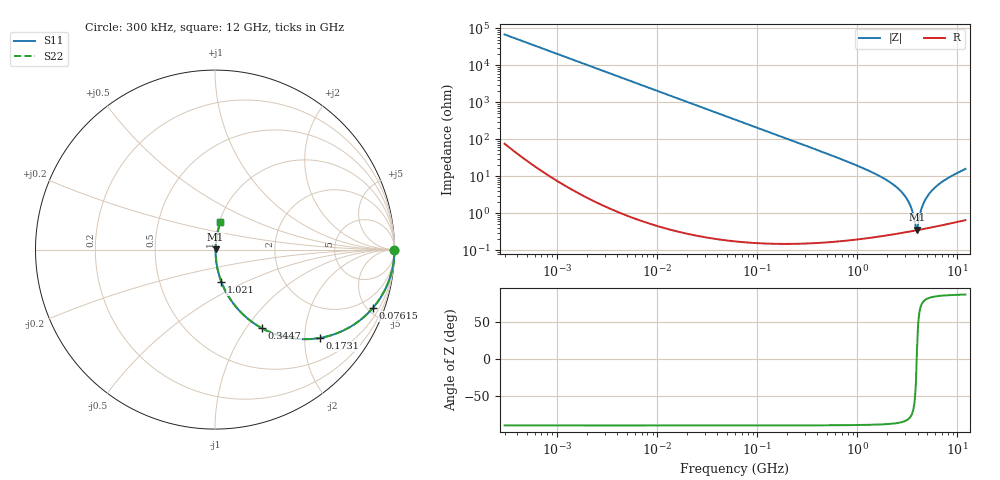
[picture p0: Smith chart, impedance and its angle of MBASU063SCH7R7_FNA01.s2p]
! MBASU063SCH7R7_FNA01  S-PARAMETER MODEL  ( General Type )
! Model Generated by TAIYO YUDEN Corporation (http://www.ty-top.com)
! Version 1.0
! TAIYO YUDEN Control No. 130801
! Copyright(c) 2013 TAIYO YUDEN CO.,LTD. All Rights Reserved.
! Product Description (link to TY-COMPAS)
! https://ds.yuden.co.jp/TYCOMPAS/or/detail?pn=MBASU063SCH7R7DFNA01&u=M
! Products Name : Multilayer Ceramic Capacitors
! Characteristics :
!  Capacitance : 7.7 pF , Rated Voltage : 50V , TCC : CH / C0H
!  Case Size : 0.6 x 0.3 / 0.024 x 0.012 [mm/inch] , Thickness : 0.3 / 0.012 [mm/inch]
!  (Conditions: Temperature = 25 degC , DC Bias Current/Voltage = 0A / 0V)
! External Node Assignments :
!  1  o---| |---o  2
! GND o---------o GND
! Frequency Range : 0.3MHz  -  12000MHz  [ 401 STEP ]
# MHz S RI R 50
! Freq[MHz].  S11 Real  S11 Imag  S21 Real  S21 Imag  S12 Real  S12 Imag  S22 Real  S22 Imag
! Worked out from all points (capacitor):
!   401 points, 300 kHz to 12 GHz, reference 50 ohm
!   read as one part in series: C = 7.73 pF near 316.3 kHz
!   lowest |Z| = 356 mohm at 3.944 GHz (marker M1)
!   series resonance near 3.917 GHz, so ESL is about 210 pH
!   S11 on the Smith chart (normalised r, x): 300 kHz: open; 76.15 MHz: 1.00, -5.41; 173.1 MHz: 1.00, -2.38; 344.7 MHz: 1.00, -1.19; 1.021 GHz: 1.00, -0.38; 12 GHz: 1.01, +0.32
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0.3  1 -0.00146  3.72e-06 0.00146  3.72e-06 0.00146  1 -0.00146
1.769972  0.9999 -0.00859  7.61e-05 0.00859  7.61e-05 0.00859  0.9999 -0.00859
10.44266  0.9974 -0.0506  0.00257 0.0506  0.00257 0.0506  0.9974 -0.0506
27.10171  0.9829 -0.1293  0.0171 0.1293  0.0171 0.1293  0.9829 -0.1293
60  0.9217 -0.2685  0.0783 0.2685  0.0783 0.2685  0.9217 -0.2685
76.15486  0.8796 -0.3252  0.1204 0.3252  0.1204 0.3252  0.8796 -0.3252
173.124  0.5851 -0.4921  0.4149 0.4921  0.4149 0.4921  0.5851 -0.4921
344.7396  0.2607 -0.4377  0.7393 0.4377  0.7393 0.4377  0.2607 -0.4377
353.9943  0.2505 -0.432  0.7495 0.432  0.7495 0.432  0.2505 -0.432
570.2811  0.1123 -0.3134  0.8877 0.3134  0.8877 0.3134  0.1123 -0.3134
1021.415  0.0359 -0.1809  0.9641 0.1809  0.9641 0.1809  0.0359 -0.1809
2088.533  0.0075 -0.07  0.9925 0.07  0.9925 0.07  0.0075 -0.07
2581.562  0.00484 -0.045  0.9952 0.045  0.9952 0.045  0.00484 -0.045
3026.31  0.00378 -0.0274  0.9962 0.0274  0.9962 0.0274  0.00378 -0.0274
3364.605  0.00345 -0.0162  0.9966 0.0162  0.9966 0.0162  0.00345 -0.0162
3740.715  0.00338 -0.00505  0.9966 0.00505  0.9966 0.00505  0.00338 -0.00505
3944.255  0.00345 0.000843  0.9966 -0.000843  0.9966 -0.000843  0.00345 0.000843
4050.141  0.00351 0.00393  0.9965 -0.00393  0.9965 -0.00393  0.00351 0.00393
4623.766  0.0041 0.0189  0.9959 -0.0189  0.9959 -0.0189  0.0041 0.0189
5565.855  0.00578 0.0406  0.9942 -0.0406  0.9942 -0.0406  0.00578 0.0406
7648.807  0.0116 0.081  0.9884 -0.081  0.9884 -0.081  0.0116 0.081
12000  0.0302 0.152  0.9698 -0.152  0.9698 -0.152  0.0302 0.152
